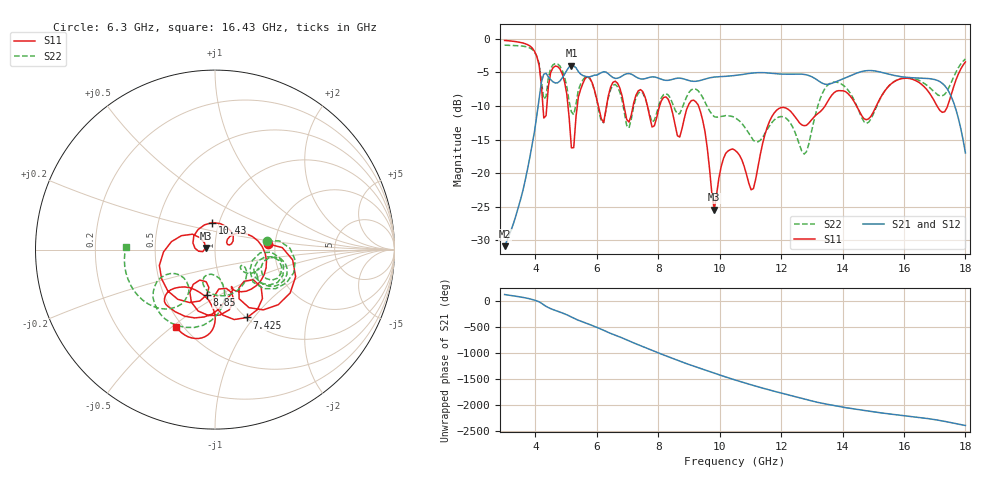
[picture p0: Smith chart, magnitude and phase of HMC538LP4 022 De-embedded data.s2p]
! Chelmsford, MA 01824
! http://www.hittite.com
! Tel: 978-250-3343
! Fax: 978-250-3373
! Device  :  HMC538LP4
! Description:  600 Analog Phase Shifter
! Frequency  :  6.0 GHz - 15.0 GHz
! Package  :  LP4  - 4x4 mm Quad Flatpack No-Lead (QFN) Plastic Package: 24 pin
! Ports  :  2 RF, 1 DC
!  Pin  3  = Rfin  = Port 1
!  Pin  16  = Rfout = Port 2
!  pin  21  = vCTL
! Voltages:  VCTL  = 0 to 5.0 Volts
! Currents :  Vb(V)  Vd(V)  Ib(mA)  Id(mA)
!  0.00  2.20  0.000000	0.472893
! Data:  The device was measured on evaluation board 111296-1.
!  Data was collected using a calibrated network analyzer.
!  The evaluation circuit board was modeled and simulated.This was use
!  to removed the evaluation board circuit from the measured data.
!  The reference plane is the center of the package pin.
! Misc:  Lot #
!Date Measured:  03 - 11 -2009
! Date:  03 - 17 -2009
! Note:
!  Hittite Microwave supplies this data as a sample of measured data at the
!  package pin for this package product.  Your particular data for this product
!  may vary.
!  Data was taken at 25 degrees C.
!  Hittite Microwave reserves the right to change this data at anytime.
# MHz S MA R 50
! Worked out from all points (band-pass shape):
!   201 points, 3 GHz to 18 GHz, reference 50 ohm
!   highest |S21| = -3.99 dB at 5.175 GHz (marker M1); lowest = -30.9 dB at 3 GHz (marker M2)
!   |S21| within 3 dB of the highest: 4.182 GHz to 17.33 GHz (13.15 GHz wide, 122 % of centre)
!   lowest |S11| = -25.4 dB at 9.825 GHz (marker M3), VSWR 1.11, Z = 45 + j0.841 ohm
!   |S11| at or under -10 dB: 8.408 GHz to 8.973 GHz (565 MHz wide, 6.5 % of centre); 9.312 GHz to 13.43 GHz (4.12 GHz wide, 36.2 % of centre); 14.46 GHz to 15.1 GHz (643.4 MHz wide, 4.35 % of centre)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
!   |S22| runs from -17.2 to -1.0 dB; largest |S21 - S12| = 0.0052
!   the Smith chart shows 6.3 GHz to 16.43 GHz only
!   S11 on the Smith chart (normalised r, x): 6.3 GHz: 1.84, +0.13; 7.425 GHz: 1.01, -0.93; 8.85 GHz: 0.81, -0.43; 10.43 GHz: 0.93, +0.29; 16.43 GHz: 0.46, -0.52
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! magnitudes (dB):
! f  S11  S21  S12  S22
! 3 GHz  -0.3  -30.9  -30.9  -1.0
! 3.975 GHz  -1.9  -13.8  -13.7  -2.0
! 4.275 GHz  -11.8  -5.3  -5.3  -9.0
! 4.8 GHz  -4.5  -6.3  -6.3  -4.1
! 5.175 GHz  -16.2  -4.0  -4.0  -10.9
! 5.55 GHz  -6.6  -5.5  -5.5  -6.1
! 6.3 GHz  -10.5  -5.0  -5.0  -10.6
! 7.425 GHz  -7.6  -6.0  -6.0  -7.9
! 8.025 GHz  -10.3  -5.9  -5.9  -9.8
! 8.85 GHz  -11.9  -6.0  -6.0  -9.5
! 9.375 GHz  -10.8  -6.2  -6.2  -8.2
! 9.825 GHz  -25.4  -5.7  -5.7  -11.6
! 10.43 GHz  -16.4  -5.5  -5.5  -11.6
! 10.5 GHz  -16.6  -5.5  -5.5  -11.7
! 11.03 GHz  -22.5  -5.1  -5.1  -14.6
! 11.78 GHz  -11.0  -5.2  -5.2  -12.1
! 13.05 GHz  -11.8  -5.8  -5.8  -12.6
! 13.65 GHz  -8.4  -6.6  -6.6  -6.5
! 15.53 GHz  -7.0  -5.3  -5.3  -6.9
! 16.43 GHz  -6.3  -5.8  -5.9  -6.1
! 17.32 GHz  -10.9  -7.0  -7.0  -8.3
! 18 GHz  -3.5  -17.0  -17.0  -3.0
